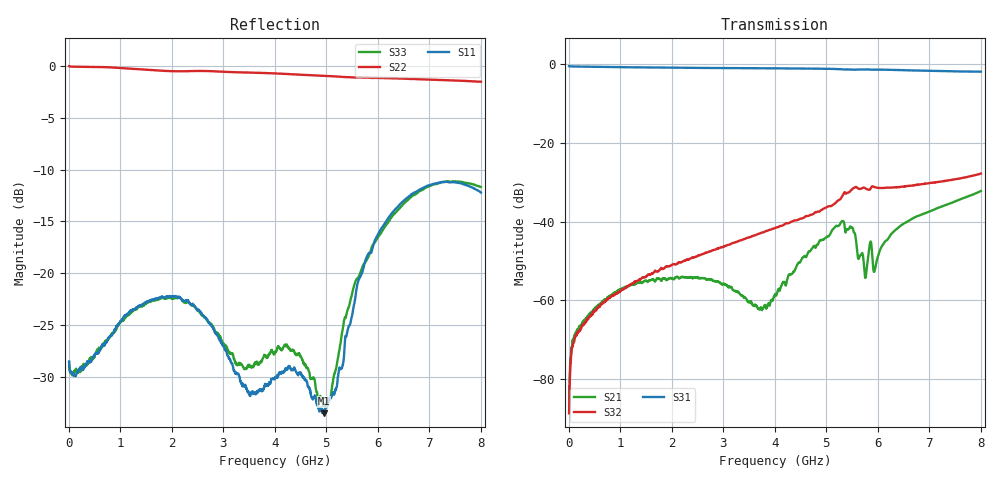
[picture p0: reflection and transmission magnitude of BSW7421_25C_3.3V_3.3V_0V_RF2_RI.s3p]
! Product: BSW7421
! Temp: 25C
! VDD: 3.300
! Control_Hi: 3.300
! Control_Lo: 0.000
! Logic State: RF2
! Port 1: RFC
! Port 2: RF1
! Port 3: RF2
! V1 = 0.00
! V2 = 0.00
! V3 = 0.00
! V4 = 0.00
# Hz S  RI  R 50
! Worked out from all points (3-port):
!   1601 points, 5 MHz to 8.005 GHz, reference 50 ohm
!   strongest paths, dB at 5 MHz, 2.005 GHz, 4.005 GHz, 6.005 GHz, 8.005 GHz:
!     S31: -0.5, -0.9, -1.1, -1.4, -1.9
!     S32: -88.7, -51.0, -41.6, -31.4, -27.8
!     S21: -88.0, -54.4, -58.5, -48.9, -32.2
!   lowest |S11| = -33.5 dB at 4.955 GHz (marker M1), VSWR 1.04, Z = 49.5 - j2.04 ohm
!   |S11| at or under -10 dB: start of sweep to end of sweep
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5000000  0.037 -0.00541  1.92e-05 4.43e-05  0.9424 -0.0133
         -2.97e-05 2.68e-05  0.9987 -0.0108  1.79e-05 2.7e-05
         0.9423 -0.0132  7.44e-06 3.61e-05  0.0367 -0.00466
8.85e8  -0.0329 -0.0419  0.00123 -0.000208  0.1157 -0.9102
        0.00124 -0.000223  0.0217 -0.9824  0.00113 0.00026
        0.116 -0.9103  0.00115 0.000233  -0.0306 -0.0426
1.805e9  -0.0443 0.0628  -4.68e-05 -0.00181  -0.8825 -0.1934
         -5.44e-05 -0.0018  -0.9487 -0.0421  0.00177 -0.00184
         -0.8826 -0.1932  0.00175 -0.00184  -0.0515 0.0561
2.85e9  0.0409 0.0309  -0.00175 0.000105  -0.0951 0.888
        -0.00175 0.000106  0.0755 0.9396  -0.00185 -0.00404
        -0.0949 0.8881  -0.00185 -0.00403  0.0336 0.0394
4.005e9  0.0274 0.0142  -0.00116 0.000169  0.8695 -0.161
         -0.00118 0.000202  0.8476 -0.3604  -0.00796 0.00226
         0.8698 -0.1615  -0.00797 0.00228  0.0361 0.0192
4.955e9  -0.00419 -0.0206  -0.00108 0.00585  -0.1298 -0.8636
         -0.00106 0.00587  -0.4471 -0.7777  -0.00108 0.0146
         -0.1302 -0.8635  -0.00109 0.0146  -0.00481 -0.0228
5.615e9  -0.0661 0.0614  0.00323 -0.00148  -0.798 -0.3061
         0.00324 -0.00148  -0.8661 0.1606  0.0242 0.0109
         -0.7979 -0.3057  0.0243 0.0108  -0.0357 0.0878
6.365e9  0.1355 0.1554  0.008 -0.000569  -0.5521 0.6373
         0.00799 -0.000595  -0.0153 0.871  0.0182 -0.0205
         -0.5522 0.6372  0.0183 -0.0205  0.1501 0.1288
7.19e9  0.2322 -0.144  0.000753 -0.0151  0.47 0.6661
        0.000686 -0.0151  0.8419 0.1569  -0.0151 -0.0283
        0.4703 0.6657  -0.0153 -0.0283  0.233 -0.1409
8.005e9  -0.0918 -0.227  -0.0242 -0.00454  0.7526 -0.279
         -0.0241 -0.00445  0.3803 -0.7489  -0.0407 0.00232
         0.7526 -0.2792  -0.0407 0.00222  -0.0325 -0.2584
